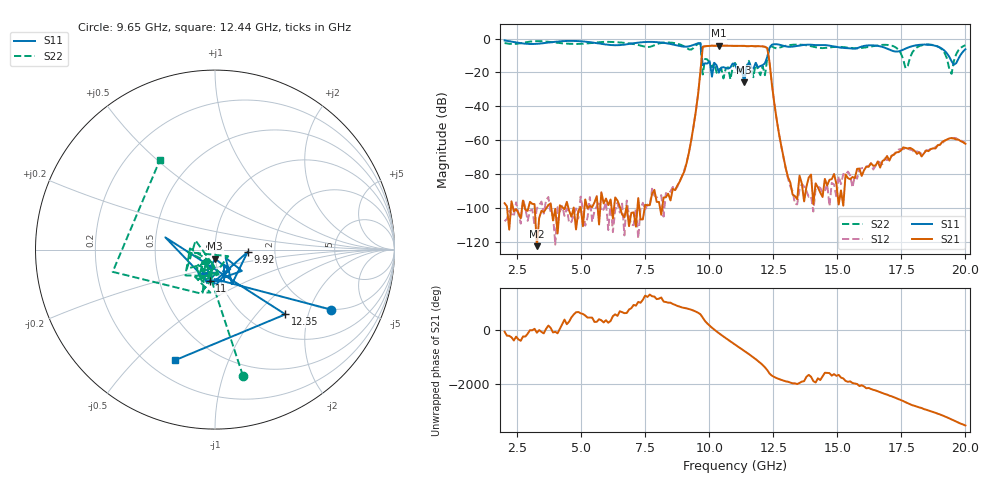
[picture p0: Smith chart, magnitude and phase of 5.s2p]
!Keysight Technologies,N5234A,MY52241180,A.10.60.03
!Date: Friday, January 20, 2023 09:33:47
!Correction: S11(Full 2 Port(1,2))
!S21(Full 2 Port(1,2))
!S12(Full 2 Port(1,2))
!S22(Full 2 Port(1,2))
!S2P File: Measurements: S11, S21, S12, S22:
# Hz S  dB  R 50
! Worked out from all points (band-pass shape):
!   201 points, 2 GHz to 20 GHz, reference 50 ohm
!   highest |S21| = -4.19 dB at 10.37 GHz (marker M1); lowest = -122.7 dB at 3.26 GHz (marker M2)
!   |S21| within 3 dB of the highest: 9.726 GHz to 12.28 GHz (2.551 GHz wide, 23.2 % of centre)
!   lowest |S11| = -25.8 dB at 11.36 GHz (marker M3), VSWR 1.11, Z = 49.9 - j5.11 ohm
!   |S11| at or under -10 dB: 9.7 GHz to 12.27 GHz (2.575 GHz wide, 23.4 % of centre); 19.33 GHz to 19.8 GHz (466.5 MHz wide, 2.38 % of centre)
!   |S22| runs from -24.2 to -1.5 dB; largest |S21 - S12| = 0.00021
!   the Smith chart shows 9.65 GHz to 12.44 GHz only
!   S11 on the Smith chart (normalised r, x): 9.65 GHz: 1.98, -2.84; 9.92 GHz: 1.44, -0.04; 11 GHz: 0.89, -0.32; 12.35 GHz: 1.43, -1.44; 12.44 GHz: 0.30, -0.66
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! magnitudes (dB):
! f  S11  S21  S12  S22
! 2 GHz  -1.1  -97.3  -108.0  -2.7
! 3.26 GHz  -3.1  -122.7  -100.2  -1.5
! 5.06 GHz  -1.7  -110.9  -100.7  -3.1
! 8.03 GHz  -2.2  -96.6  -92.8  -2.9
! 9.02 GHz  -4.8  -78.5  -77.6  -4.7
! 9.65 GHz  -2.7  -19.5  -19.5  -2.9
! 9.74 GHz  -15.7  -4.9  -4.9  -21.2
! 9.92 GHz  -14.8  -4.4  -4.4  -12.4
! 10.37 GHz  -20.2  -4.2  -4.2  -18.4
! 11 GHz  -15.0  -4.3  -4.3  -14.4
! 11.36 GHz  -25.8  -4.3  -4.3  -22.9
! 11.54 GHz  -14.1  -4.5  -4.5  -13.2
! 12.17 GHz  -14.6  -4.9  -4.9  -21.7
! 12.35 GHz  -5.5  -14.1  -14.1  -4.7
! 12.44 GHz  -3.7  -26.9  -26.9  -4.6
! 13.07 GHz  -4.8  -81.9  -82.7  -4.0
! 14.06 GHz  -3.8  -97.9  -102.2  -4.8
! 17.03 GHz  -6.5  -72.1  -70.3  -3.9
! 17.66 GHz  -6.0  -64.6  -64.6  -17.5
! 18.92 GHz  -4.8  -63.1  -63.1  -4.7
! 19.46 GHz  -13.4  -58.8  -59.1  -20.9
! 20 GHz  -6.4  -62.2  -61.6  -4.0
